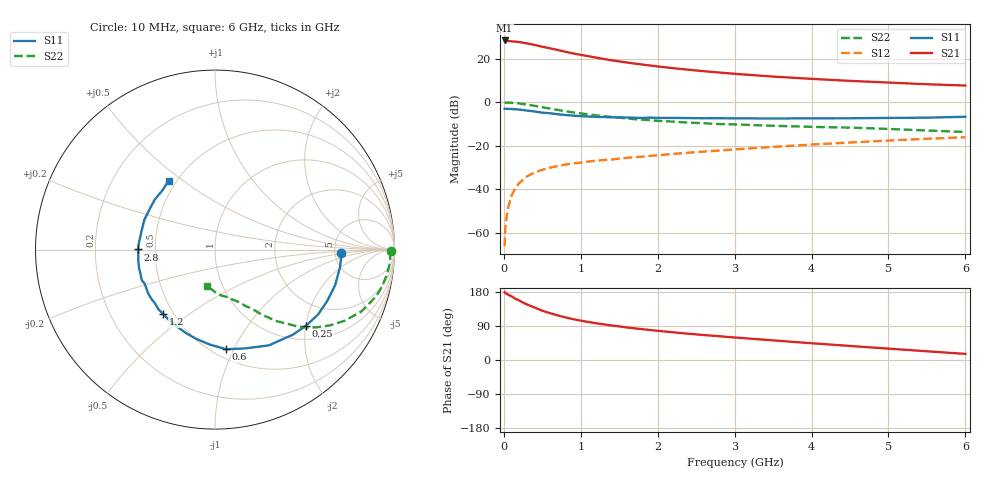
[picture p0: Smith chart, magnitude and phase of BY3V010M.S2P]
! SIEMENS Small Signal Semiconductors
! BFY420
! Si NPN RF SIEGET Grounded Emitter Transistor in MICRO-X
! VCE = 3 V  IC = 10 mA
! Common Emitter S-Parameters:  October  1996
# GHz  S  MA  R  50
!  f  S11  S21  S12  S22
! GHz  MAG  ANG  MAG  ANG  MAG  ANG  MAG  ANG
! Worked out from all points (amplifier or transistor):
!   36 points, 10 MHz to 6 GHz, reference 50 ohm
!   highest |S21| = 28.3 dB at 10 MHz (marker M1)
!   |S21| within 3 dB of that: start of sweep to 515.2 MHz
!   unconditionally stable (mu >= 1): 2.525 GHz to end of sweep
!   at 250 MHz: K = 0.20, MSG = 31.4 dB, |S12| = -35.5 dB
!   at 1.4 GHz: K = 0.75, MSG = 22.7 dB, |S12| = -26.3 dB
!   at 6 GHz: K = 1.09, MAG = 10.0 dB, |S12| = -16.1 dB
!   S11 on the Smith chart (normalised r, x): 10 MHz: 5.71, -0.47; 250 MHz: 1.34, -2.01; 600 MHz: 0.58, -0.93; 1.2 GHz: 0.44, -0.40; 2.8 GHz: 0.40, +0.00; 6 GHz: 0.45, +0.44
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0.01  0.7038 -1.7  26.04 179.0  0.0005 80.5  0.9795 -0.6
0.02  0.7038 -3.6  25.86 176.6  0.0014 83.4  0.9757 -1.4
0.05  0.7035 -8.0  25.24 173.2  0.0035 82.6  0.979 -4.0
0.1  0.6981 -16.5  24.93 168.2  0.0072 82.5  0.9684 -8.2
0.15  0.6878 -24.6  24.4 161.6  0.0108 76.0  0.9538 -12.3
0.2  0.6785 -32.3  23.86 157.1  0.014 74.3  0.9365 -15.9
0.25  0.6611 -39.8  23.12 151.5  0.0167 70.4  0.9089 -19.5
0.3  0.6432 -47.4  22.29 146.6  0.0199 68.9  0.8853 -22.9
0.4  0.612 -60.7  20.58 138.4  0.0245 63.5  0.8244 -28.7
0.5  0.5754 -73.1  18.67 130.0  0.0281 59.8  0.767 -33.4
0.6  0.5584 -83.6  17.18 123.7  0.0316 57.6  0.7142 -37.3
0.8  0.5085 -101.8  14.35 112.4  0.0372 52.8  0.6229 -43.3
0.9  0.4928 -109.0  13.14 107.8  0.0397 51.7  0.5847 -45.3
1.1  0.4689 -123.1  11.34 100.3  0.0436 50.7  0.5255 -49.3
1.2  0.4612 -128.6  10.54 96.9  0.0457 50.3  0.4995 -50.8
1.6  0.4454 -146.7  8.122 85.8  0.0529 48.9  0.423 -55.7
2.2  0.4358 -165.7  6.019 73.1  0.0652 48.4  0.3581 -61.5
2.8  0.4291 179.9  4.792 62.7  0.0777 46.9  0.3156 -66.5
3.5  0.422 166.1  3.867 51.8  0.0944 44.2  0.2877 -72.0
4.5  0.4282 148.6  3.082 37.1  0.119 38.3  0.2615 -81.0
5.5  0.4418 131.3  2.58 23.0  0.1449 30.6  0.2245 -94.1
6  0.4634 123.9  2.411 16.1  0.1573 26.3  0.2075 -102.7
